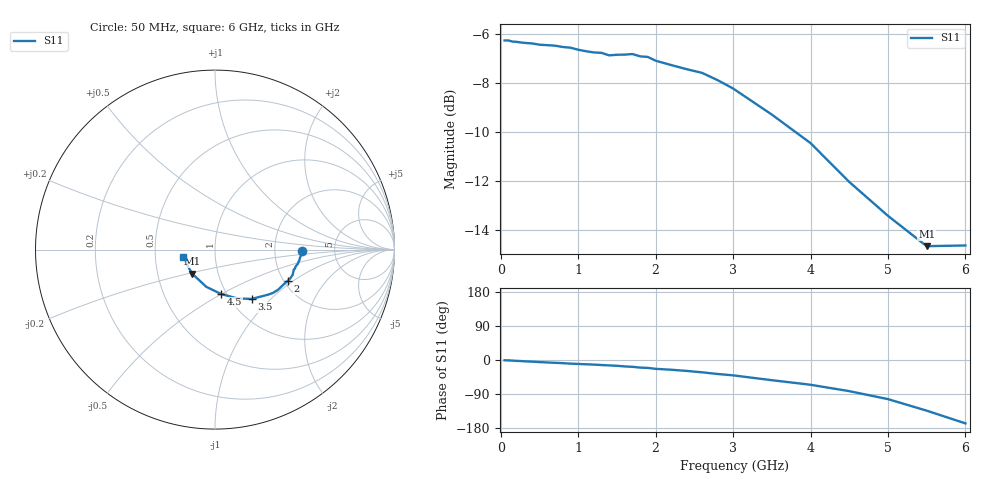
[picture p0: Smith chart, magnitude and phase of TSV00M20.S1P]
! SIEMENS Small Signal Semiconductors
! BAT14-03W
! Si Schottky Diode in SOD323
! IF = 0.2 mA
! S-Parameters:  November  1995
# GHz  S  MA  R  50
!  f  S11
! GHz  MAG  ANG
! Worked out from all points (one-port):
!   34 points, 50 MHz to 6 GHz, reference 50 ohm
!   lowest |S11| = -14.7 dB at 5.5 GHz (marker M1), VSWR 1.45, Z = 37.5 - j10.4 ohm
!   |S11| at or under -10 dB: 3.799 GHz to end of sweep
!   S11 on the Smith chart (normalised r, x): 50 MHz: 2.88, -0.04; 2 GHz: 2.10, -0.91; 3.5 GHz: 1.25, -0.78; 4.5 GHz: 0.94, -0.50; 6 GHz: 0.69, -0.06
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0.05  0.4852 -0.7
0.1  0.4852 -1.0
0.2  0.4821 -2.3
0.25  0.4808 -2.7
0.5  0.4756 -5.5
0.7  0.4735 -7.4
0.8  0.4705 -8.3
0.9  0.469 -9.6
1.2  0.4586 -12.1
1.3  0.4578 -13.3
1.4  0.4524 -14.3
1.5  0.4537 -15.3
1.6  0.4539 -16.9
1.7  0.4553 -18.0
1.8  0.4503 -20.0
1.9  0.449 -20.9
2  0.4411 -23.3
2.2  0.4323 -25.7
2.4  0.4239 -28.8
2.6  0.4167 -32.5
2.8  0.4027 -36.9
3  0.3872 -40.5
3.5  0.3426 -53.3
4  0.2997 -65.3
4.5  0.2497 -82.2
5  0.213 -103.2
5.5  0.1847 -133.7
6  0.1853 -167.2
